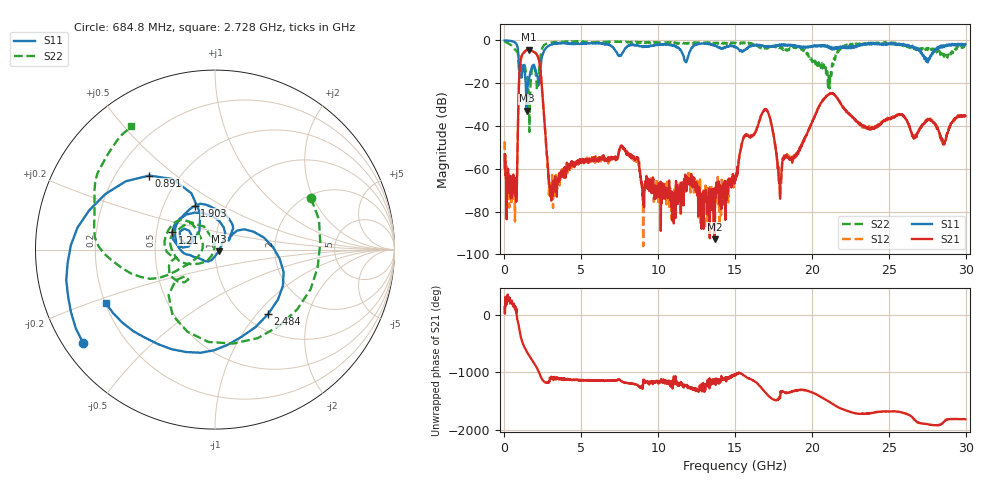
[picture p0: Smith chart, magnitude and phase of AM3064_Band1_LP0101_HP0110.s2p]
# Hz S DB R 50.0
!freq dBS11 angS11 dBS21 angS21 dBS12 angS12 dBS22 angS22
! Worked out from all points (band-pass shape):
!   1600 points, 10 MHz to 29.98 GHz, reference 50 ohm
!   highest |S21| = -4.37 dB at 1.584 GHz (marker M1); lowest = -93.0 dB at 13.67 GHz (marker M2)
!   |S21| within 3 dB of the highest: 1.115 GHz to 2.163 GHz (1.048 GHz wide, 63.9 % of centre)
!   lowest |S11| = -32.9 dB at 1.435 GHz (marker M3), VSWR 1.05, Z = 52.1 - j0.939 ohm
!   |S11| at or under -10 dB: 931.5 MHz to 2.388 GHz (1.456 GHz wide, 87.7 % of centre); 11.7858 GHz to 11.83811 GHz (52.31 MHz wide, 0.443 % of centre); 27.52327 GHz to 27.55143 GHz (28.16 MHz wide, 0.102 % of centre)
!   |S22| runs from -42.8 to -0.4 dB; largest |S21 - S12| = 0.0095
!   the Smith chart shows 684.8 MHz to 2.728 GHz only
!   S11 on the Smith chart (normalised r, x): 684.8 MHz: 0.06, -0.32; 891 MHz: 0.34, +0.41; 1.21 GHz: 0.60, +0.12; 1.903 GHz: 0.72, +0.38; 2.484 GHz: 1.25, -1.15; 2.728 GHz: 0.20, -0.22
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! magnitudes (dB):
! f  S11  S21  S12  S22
! 10 MHz  0.0  -53.2  -47.3  -0.4
! 684.8 MHz  -0.9  -72.5  -84.7  -4.3
! 891 MHz  -5.2  -35.1  -35.2  -7.2
! 1.21 GHz  -11.8  -6.1  -6.1  -11.0
! 1.435 GHz  -32.9  -4.6  -4.5  -16.5
! 1.584 GHz  -18.4  -4.4  -4.4  -26.5
! 1.903 GHz  -11.4  -5.4  -5.3  -11.9
! 2.484 GHz  -6.6  -26.4  -26.3  -3.3
! 2.728 GHz  -3.4  -50.3  -50.3  -1.6
! 3.046 GHz  -1.9  -75.0  -71.8  -1.0
! 5.015 GHz  -1.4  -56.7  -55.9  -0.7
! 7.657 GHz  -6.0  -49.6  -49.4  -0.7
! 10 GHz  -2.0  -71.2  -70.2  -0.9
! 13.67 GHz  -2.5  -93.0  -73.6  -1.2
! 15 GHz  -3.1  -63.5  -62.9  -1.3
! 16.92 GHz  -2.8  -32.2  -32.4  -3.7
! 17.91 GHz  -2.0  -71.8  -67.2  -3.2
! 19.99 GHz  -3.1  -38.6  -38.5  -9.3
! 21.27 GHz  -3.3  -24.8  -24.7  -16.5
! 25 GHz  -1.3  -36.9  -36.3  -1.2
! 28.54 GHz  -2.3  -47.8  -48.2  -6.2
! 29.98 GHz  -1.8  -35.3  -35.3  -2.9
